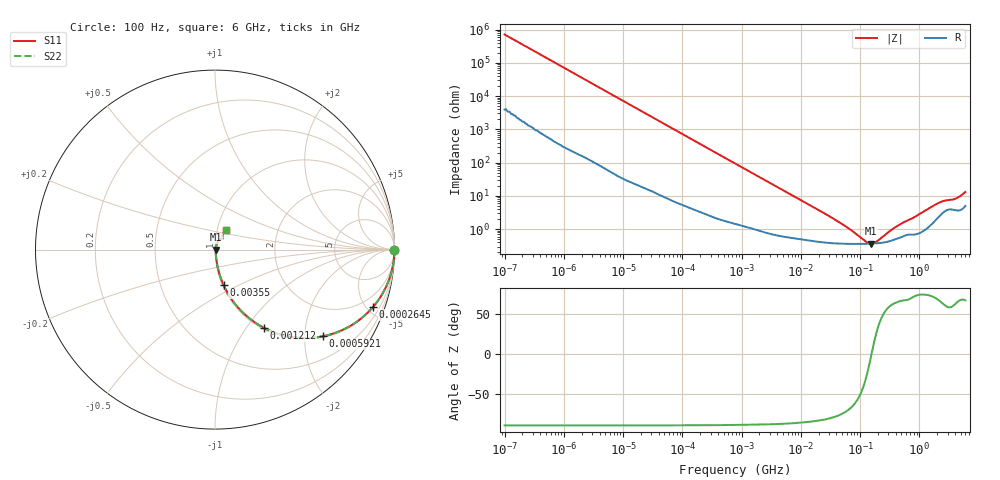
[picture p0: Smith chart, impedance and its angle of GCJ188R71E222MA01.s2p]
!Murata Part Number: GCJ188R71E222MA01
!These Parameters are Measured in Series Mode Connection
!Data Generated on Mar 13, 2026
!  o--ll--o
!Port1  Port2
!  o------o
!Operation Temp=25[degC], DC Bias Voltage=0[V]
!Freq. Start=100[Hz] Stop=6[GHz] 401[Steps]
# Hz S RI R 50
!Freq.(Hz) S11(Real) S11(Imag) S21(Real) S21(Imag) S12(Real) S12(Imag) S22(Real) S22(Imag)
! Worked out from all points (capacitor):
!   401 points, 100 Hz to 6 GHz, reference 50 ohm
!   read as one part in series: C = 2.24 nF near 109 Hz
!   lowest |Z| = 369 mohm at 152.6 MHz (marker M1)
!   series resonance near 156 MHz, so ESL is about 460 pH
!   S11 on the Smith chart (normalised r, x): 100 Hz: open; 264.5 kHz: 1.05, -5.50; 592.1 kHz: 1.03, -2.47; 1.212 MHz: 1.02, -1.21; 3.55 MHz: 1.01, -0.42; 6 GHz: 1.10, +0.24
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100  1 -0.000141  8e-07 0.000141  8e-07 0.000141  1 -0.000141
2008  1 -0.00281  2.04e-05 0.00281  2.04e-05 0.00281  1 -0.00281
40335  0.9966 -0.0557  0.00345 0.0557  0.00345 0.0557  0.9966 -0.0557
108014  0.9772 -0.1455  0.0228 0.1455  0.0228 0.1455  0.9772 -0.1455
264476  0.8809 -0.319  0.1191 0.319  0.1191 0.319  0.8809 -0.319
395726  0.7699 -0.4154  0.2301 0.4154  0.2301 0.4154  0.7699 -0.4154
592111  0.6022 -0.4828  0.3978 0.4828  0.3978 0.4828  0.6022 -0.4828
774597  0.4721 -0.4916  0.5279 0.4916  0.5279 0.4916  0.4721 -0.4916
1212075  0.2726 -0.4357  0.7274 0.4357  0.7274 0.4357  0.2726 -0.4357
1983483  0.1276 -0.3218  0.8724 0.3218  0.8724 0.3218  0.1276 -0.3218
3549919  0.0478 -0.1977  0.9522 0.1977  0.9522 0.1977  0.0478 -0.1977
1.555665e7  0.00669 -0.0477  0.9933 0.0477  0.9933 0.0477  0.00669 -0.0477
5.211241e7  0.00382 -0.013  0.9962 0.013  0.9962 0.013  0.00382 -0.013
1.275994e8  0.00364 -0.00198  0.9964 0.00198  0.9964 0.00198  0.00364 -0.00198
1.526266e8  0.00367 -0.000213  0.9963 0.000213  0.9963 0.000213  0.00367 -0.000213
1.909225e8  0.00377 0.002  0.9962 -0.002  0.9962 -0.002  0.00377 0.002
3.124326e8  0.00438 0.0074  0.9956 -0.0074  0.9956 -0.0074  0.00438 0.0074
4.888888e8  0.00582 0.0132  0.9942 -0.0132  0.9942 -0.0132  0.00582 0.0132
1.95892e9  0.0223 0.0517  0.9777 -0.0517  0.9777 -0.0517  0.0223 0.0517
2.562649e9  0.0348 0.0587  0.9652 -0.0587  0.9652 -0.0587  0.0348 0.0587
4.009986e9  0.0407 0.067  0.9593 -0.067  0.9593 -0.067  0.0407 0.067
6e9  0.0602 0.1086  0.9398 -0.1086  0.9398 -0.1086  0.0602 0.1086
